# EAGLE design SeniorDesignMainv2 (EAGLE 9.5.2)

## Sheet 1 of 5: ESP32 Pinout and Power In ESP32 Device Pinout with connections to all other devices
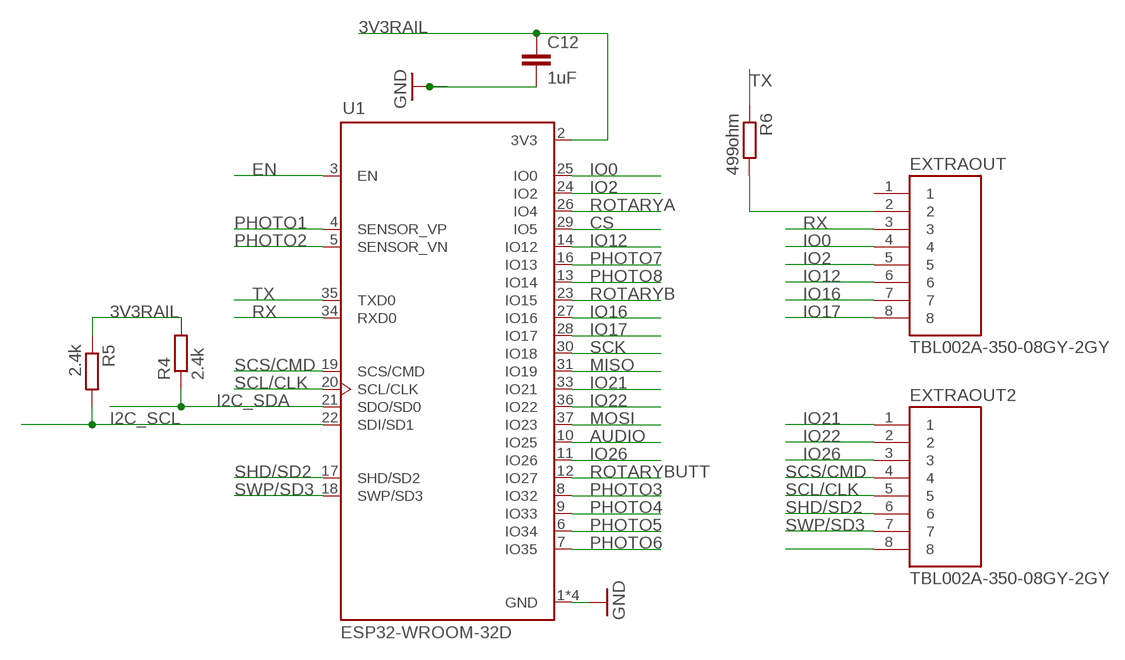
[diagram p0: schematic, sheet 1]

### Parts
C12  1uF  C-EUC1206  [C1206]
EXTRAOUT  TBL002A-350-08GY-2GY  [CUI_TBL002A-350-08GY-2GY]
EXTRAOUT2  TBL002A-350-08GY-2GY  [CUI_TBL002A-350-08GY-2GY]
R4  2.4k  R-EU_R1206  [R1206]
R5  2.4k  R-EU_R1206  [R1206]
R6  499ohm  R-EU_R1206  [R1206]
U1  ESP32-WROOM-32D  [MODULE_ESP32-WROOM-32D]

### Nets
3V3RAIL: C12.1 R4.2 R5.1 U1.2(3V3) ; also sheet 2,4,5
AUDIO: U1.10(IO25) ; also sheet 3
CS: U1.29(IO5) ; also sheet 5
EN: U1.3(EN)
GND: C12.2 U1.1(GND) U1.15(GND) U1.38(GND) U1.39(GND) ; also sheet 2,3,4,5
I2C_SCL: R5.2 U1.22(SDI/SD1) ; also sheet 5
I2C_SDA: R4.1 U1.21(SDO/SD0) ; also sheet 5
IO0: EXTRAOUT.4 U1.25(IO0)
IO2: EXTRAOUT.5 U1.24(IO2)
IO12: EXTRAOUT.6 U1.14(IO12)
IO16: EXTRAOUT.7 U1.27(IO16)
IO17: EXTRAOUT.8 U1.28(IO17)
IO21: EXTRAOUT2.1 U1.33(IO21)
IO22: EXTRAOUT2.2 U1.36(IO22)
IO26: EXTRAOUT2.3 U1.11(IO26)
MISO: U1.31(IO19) ; also sheet 5
MOSI: U1.37(IO23) ; also sheet 5
N$8: EXTRAOUT.2 R6.2
N$12: EXTRAOUT2.8
PHOTO1: U1.4(SENSOR_VP) ; also sheet 4
PHOTO2: U1.5(SENSOR_VN) ; also sheet 4
PHOTO3: U1.8(IO32) ; also sheet 4
PHOTO4: U1.9(IO33) ; also sheet 4
PHOTO5: U1.6(IO34) ; also sheet 4
PHOTO6: U1.7(IO35) ; also sheet 4
PHOTO7: U1.16(IO13) ; also sheet 4
PHOTO8: U1.13(IO14) ; also sheet 4
ROTARYA: U1.26(IO4) ; also sheet 5
ROTARYB: U1.23(IO15) ; also sheet 5
ROTARYBUTT: U1.12(IO27) ; also sheet 5
RX: EXTRAOUT.3 U1.34(RXD0)
SCK: U1.30(IO18) ; also sheet 5
SCL/CLK: EXTRAOUT2.5 U1.20(SCL/CLK)
SCS/CMD: EXTRAOUT2.4 U1.19(SCS/CMD)
SHD/SD2: EXTRAOUT2.6 U1.17(SHD/SD2)
SWP/SD3: EXTRAOUT2.7 U1.18(SWP/SD3)
TX: R6.1 U1.35(TXD0)
Unconnected: EXTRAOUT.1

## Sheet 2 of 5: Power/Voltage Regulators Basic/per data sheet setups for all the voltage regulators
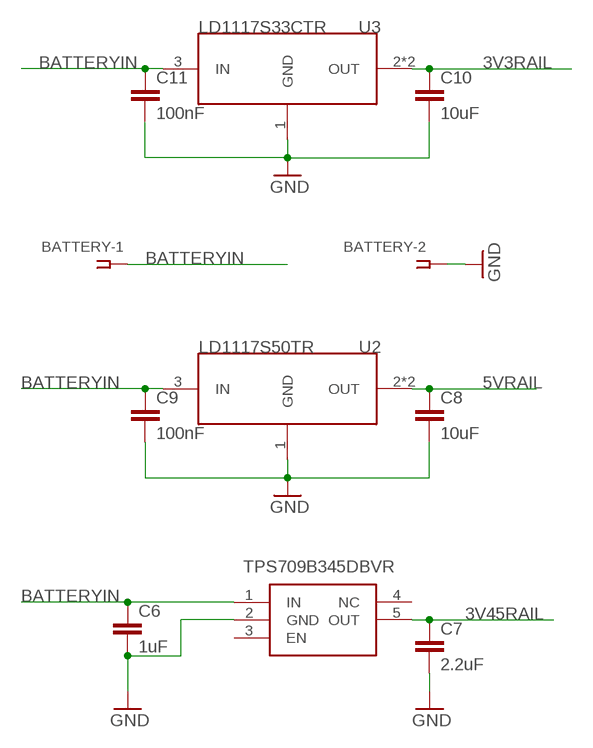
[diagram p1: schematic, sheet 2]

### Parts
BATTERY  SSW-101-02-G-D  [SSW-101-02-G-D]
C6  1uF  C-EUC1206  [C1206]
C7  2.2uF  C-EUC1206  [C1206]
C8  10uF  C-EUC1206  [C1206]
C9  100nF  C-EUC1206  [C1206]
C10  10uF  C-EUC1206  [C1206]
C11  100nF  C-EUC1206  [C1206]
IC1  TPS709B345DBVR  [SOT95P280X145-5N]
U2  LD1117S50TR  [SOT223]
U3  LD1117S33CTR  [SOT223]

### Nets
3V3RAIL: C10.1 U3.2(OUT) U3.4(OUT) ; also sheet 1,4,5
3V45RAIL: C7.1 IC1.5(OUT) ; also sheet 4
5VRAIL: C8.1 U2.2(OUT) U2.4(OUT) ; also sheet 3,5
BATTERYIN: BATTERY.1 C6.1 C9.1 C11.1 IC1.1(IN) U2.3(IN) U3.3(IN)
GND: BATTERY.2 C6.2 C7.2 C8.2 C9.2 C10.2 C11.2 IC1.2(GND) U2.1(GND) U3.1(GND) ; also sheet 1,3,4,5
Unconnected: IC1.3(EN) IC1.4(NC)

## Sheet 3 of 5: Audio Circuit LM 386 with Bass Boost Requires: 5 Capacitors, 3 Resistors, 4 Mount Holes
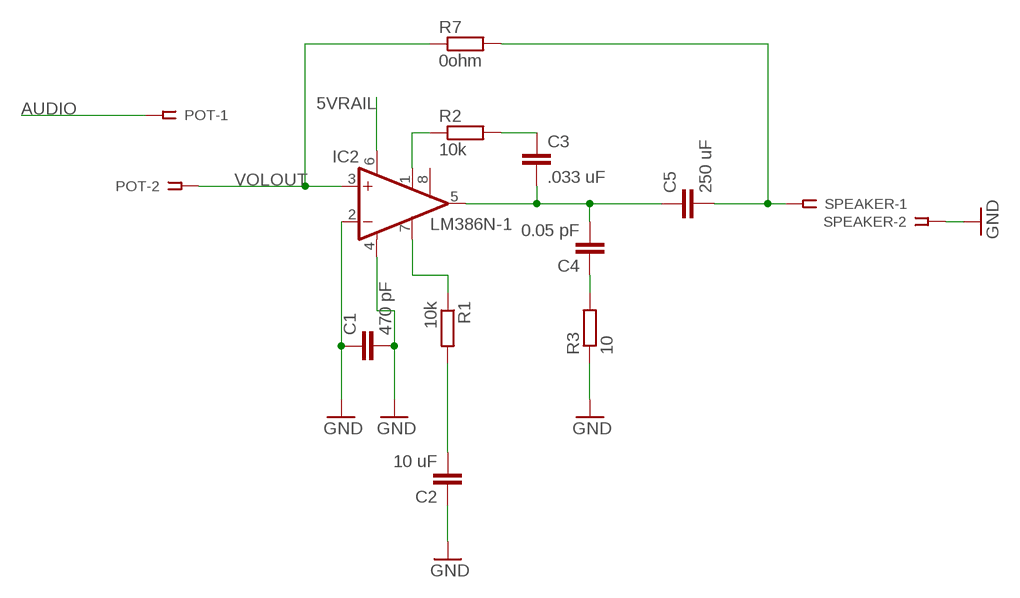
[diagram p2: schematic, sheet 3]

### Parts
C1  470 pF  C-EUC1206  [C1206]
C2  10 uF  C-EUC1206  [C1206]
C3  .033 uF  C-EUC1206  [C1206]
C4  0.05 pF  C-EUC1206  [C1206]
C5  250 uF  C-EUC1206  [C1206]
IC2  LM386N-1  [DIL08]
POT  SSW-101-02-G-D  [SSW-101-02-G-D]
R1  10k  R-EU_R1206  [R1206]
R2  10k  R-EU_R1206  [R1206]
R3  10  R-EU_R1206  [R1206]
R7  0ohm  R-EU_R1206  [R1206]
SPEAKER  SSW-101-02-G-D  [SSW-101-02-G-D]

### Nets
5VRAIL: IC2.6(VS) ; also sheet 2,5
AUDIO: POT.1 ; also sheet 1
GND: C1.1 C1.2 C2.1 IC2.2(-IN) IC2.4(GND) R3.1 SPEAKER.2 ; also sheet 1,2,4,5
N$1: IC2.7(BYPASS) R1.1
N$2: C2.2 R1.2
N$3: IC2.1(GAIN) R2.1
N$4: C3.2 C4.2 C5.1 IC2.5(OUT)
N$5: C3.1 R2.2
N$6: C4.1 R3.2
N$7: C5.2 R7.2 SPEAKER.1
VOLOUT: IC2.3(+IN) POT.2 R7.1
Unconnected: IC2.8(GAIN)

## Sheet 4 of 5: Laser Diodes and Photo Transistors Mapping from MCU to ports for the laser diodes. Mapping from MCU to ports for the phototransistors. WARNING: MCU LINES AND PORT HOLES ARE 1 INDEXED Extra Terminal for ground connections
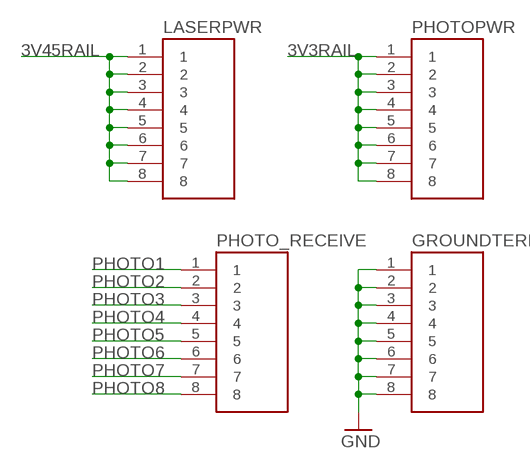
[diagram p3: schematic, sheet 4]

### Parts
GROUNDTERM  TBL002A-350-08GY-2GY  [CUI_TBL002A-350-08GY-2GY]
LASERPWR  TBL002A-350-08GY-2GY  [CUI_TBL002A-350-08GY-2GY]
PHOTO_RECEIVE  TBL002A-350-08GY-2GY  [CUI_TBL002A-350-08GY-2GY]
PHOTOPWR  TBL002A-350-08GY-2GY  [CUI_TBL002A-350-08GY-2GY]

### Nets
3V3RAIL: PHOTOPWR.1 PHOTOPWR.2 PHOTOPWR.3 PHOTOPWR.4 PHOTOPWR.5 PHOTOPWR.6 PHOTOPWR.7 PHOTOPWR.8 ; also sheet 1,2,5
3V45RAIL: LASERPWR.1 LASERPWR.2 LASERPWR.3 LASERPWR.4 LASERPWR.5 LASERPWR.6 LASERPWR.7 LASERPWR.8 ; also sheet 2
GND: GROUNDTERM.1 GROUNDTERM.2 GROUNDTERM.3 GROUNDTERM.4 GROUNDTERM.5 GROUNDTERM.6 GROUNDTERM.7 GROUNDTERM.8 ; also sheet 1,2,3,5
PHOTO1: PHOTO_RECEIVE.1 ; also sheet 1
PHOTO2: PHOTO_RECEIVE.2 ; also sheet 1
PHOTO3: PHOTO_RECEIVE.3 ; also sheet 1
PHOTO4: PHOTO_RECEIVE.4 ; also sheet 1
PHOTO5: PHOTO_RECEIVE.5 ; also sheet 1
PHOTO6: PHOTO_RECEIVE.6 ; also sheet 1
PHOTO7: PHOTO_RECEIVE.7 ; also sheet 1
PHOTO8: PHOTO_RECEIVE.8 ; also sheet 1

## Sheet 5 of 5: SPI to SD, I2C to LCD SD - Routing the MCU to communicate to the SD Card Reader via SPI potocol. The connection seen here is to a 7 pin header that will be on the board. This is the connection point for the breakout board and the MCU. LCD - 4 Pin Header. This could be to either a module for I2C or the chip if it's an issue to use the I2C module. 5 V are needed for the module and LCD. The 5 V Rail could be a direct connection from 5 V regulator or it could be from this pin.
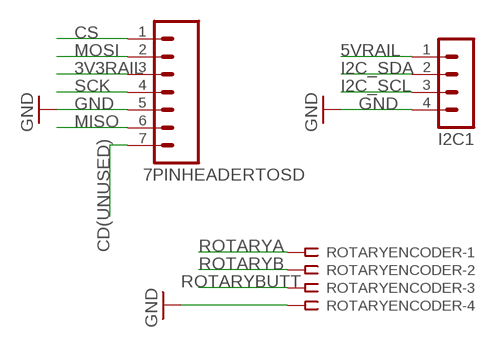
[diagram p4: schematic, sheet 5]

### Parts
7PINHEADERTOSD  M07  [07P]
I2C1  MA04-1  [MA04-1]
ROTARYENCODER  SSW-104-02-G-S  [SSW-104-02-G-S]

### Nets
3V3RAIL: 7PINHEADERTOSD.3 ; also sheet 1,2,4
5VRAIL: I2C1.1 ; also sheet 2,3
CD(UNUSED): 7PINHEADERTOSD.7
CS: 7PINHEADERTOSD.1 ; also sheet 1
GND: 7PINHEADERTOSD.5 I2C1.4 ROTARYENCODER.4 ; also sheet 1,2,3,4
I2C_SCL: I2C1.3 ; also sheet 1
I2C_SDA: I2C1.2 ; also sheet 1
MISO: 7PINHEADERTOSD.6 ; also sheet 1
MOSI: 7PINHEADERTOSD.2 ; also sheet 1
ROTARYA: ROTARYENCODER.1 ; also sheet 1
ROTARYB: ROTARYENCODER.2 ; also sheet 1
ROTARYBUTT: ROTARYENCODER.3 ; also sheet 1
SCK: 7PINHEADERTOSD.4 ; also sheet 1

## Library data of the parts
7PINHEADERTOSD = con-amp-quick:M07: AMP QUICK CONNECTOR; OC_FARNELL: unknown; OC_NEWARK: unknown
BATTERY POT SPEAKER = con-samtec:SSW-101-02-G: THROUGH-HOLE .025" SQ POST SOCKET; MF: Samtec Inc.; MPN: SSW-101-02-G-D; OC_FARNELL: unknown; OC_NEWARK: 82P1456
C1-C12 = rcl:C-EU: CAPACITOR, European symbol; SPICEPREFIX: C
EXTRAOUT EXTRAOUT2 GROUNDTERM LASERPWR PHOTO_RECEIVE PHOTOPWR = TBL002A-350-08GY-2GY:TBL002A-350-08GY-2GY; AVAILABILITY: Unavailable; CUI_PURCHASE_URL: https://www.cuidevices.com/product/interconnect/connectors/terminal-blocks/tbl002a-350-series?utm_source=snapeda.com&utm_medium=referral&utm_campaign=snapedaBOM; DESCRIPTION: 1~24 Poles, Screwless, 45°, 3.50 Pitch, 24~20 _AWG_, Terminal Block Connector; MF: CUI Devices; MP: TBL002A-350-08GY-2GY; PACKAGE: None; PRICE: None
I2C1 = con-lstb:MA04-1: PIN HEADER; OC_FARNELL: unknown; OC_NEWARK: unknown
IC1 = SamacSys_Parts:TPS709B345DBVR: LDO Voltage Regulators TPS709 DIE IN TLV704 PINOUT Source: Datasheet; DESCRIPTION: LDO Voltage Regulators TPS709 DIE IN TLV704 PINOUT; HEIGHT: 1.45mm; MANUFACTURER_NAME: Texas Instruments; MANUFACTURER_PART_NUMBER: TPS709B345DBVR
IC2 = linear:LM386?-*: Low Voltage Audio Power Amplifier Source: http://cache.national.com/ds/LM/LM386.pdf
R1-R7 = rcl:R-EU_: RESISTOR, European symbol; SPICEPREFIX: R
ROTARYENCODER = con-samtec:SSW-104-02-G-S: THROUGH-HOLE .025" SQ POST SOCKET Source: Samtec SSW.pdf; MF: Samtec Inc.; MPN: SSW-104-02-G-S; OC_FARNELL: unknown; OC_NEWARK: 11P9384
U1 = ESP32-WROOM-32D:ESP32-WROOM-32D: IC: SoC; GPIO, I2C, I2S, IR, SD, SDIO, SPI, UART; 2.7÷3.6VDC; 20dBm; AVAILABILITY: Unavailable; DESCRIPTION: Bluetooth, WiFi 802.11b/g/n, Bluetooth v4.2 + EDR, Class 1, 2 and 3 Transceiver Module 2.4GHz ~ 2.5GHz Integrated, Trace Surface Mount; MF: Espressif Systems; MP: ESP32-WROOM-32D; PACKAGE: Module Espressif Systems; PRICE: None
U2 = LD1117S50TR:LD1117S50TR: http://octopart.com/ld1117s50tr-stmicroelectronics-529395; AVAILABILITY: Unavailable; DESCRIPTION: Linear Voltage Regulator IC 1 Output 800mA SOT-223; MF: STMicroelectronics; MP: LD1117S50TR; PACKAGE: SOT-223 STMicroelectronics; PRICE: None
U3 = LD1117S33CTR:LD1117S33CTR: http://octopart.com/ld1117s33tr-stmicroelectronics-526708; AVAILABILITY: Unavailable; DESCRIPTION: Linear Voltage Regulator IC 1 Output 800mA SOT-223; MF: STMicroelectronics; MP: LD1117S33CTR; PACKAGE: SOT-223 STMicroelectronics; PRICE: None

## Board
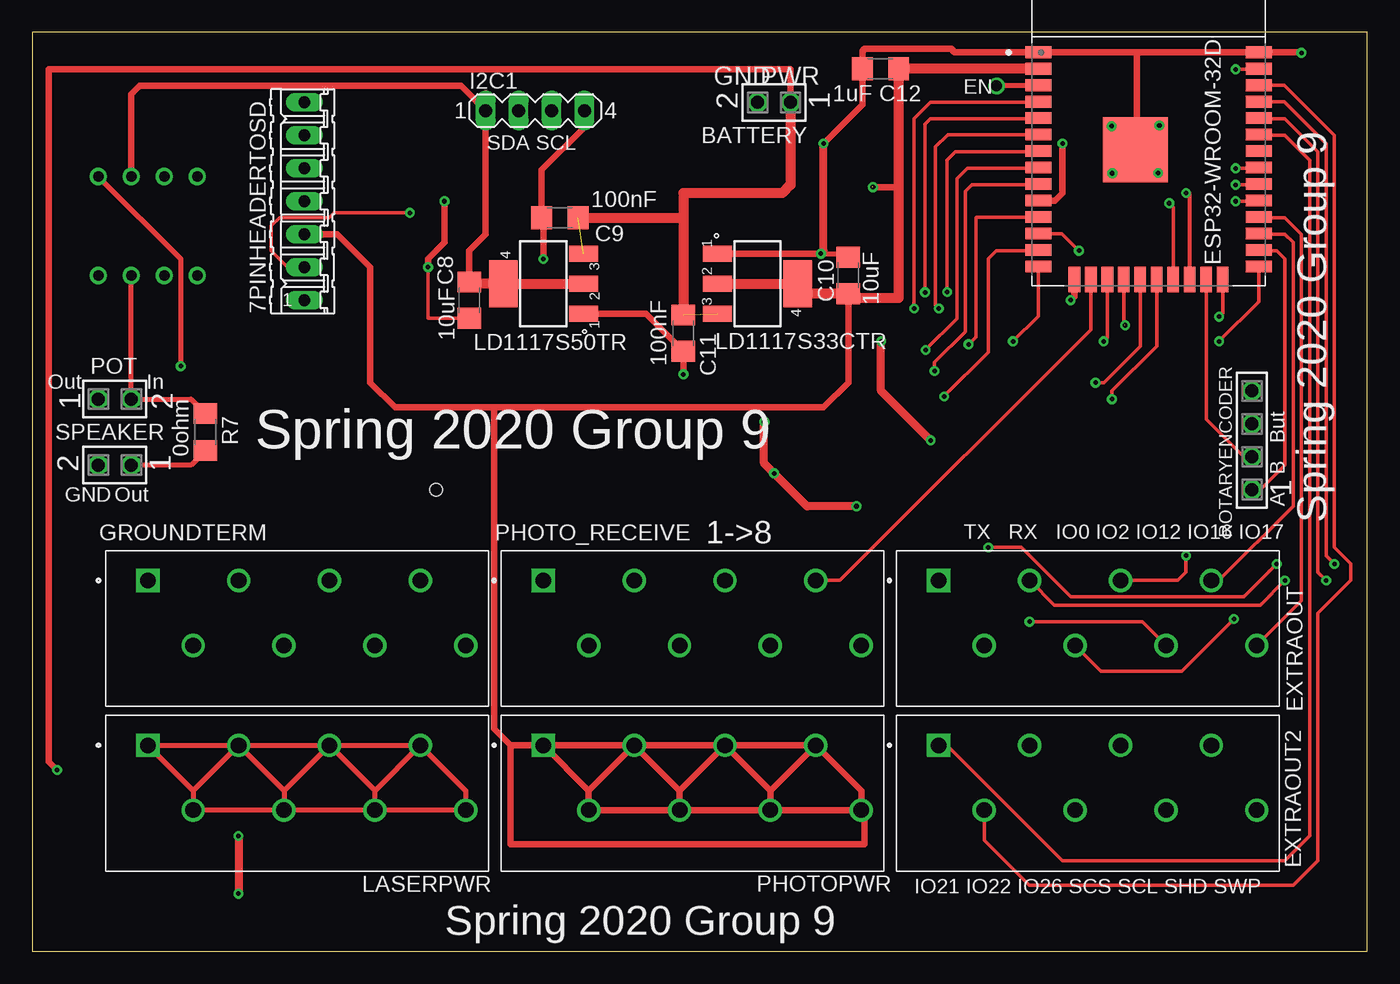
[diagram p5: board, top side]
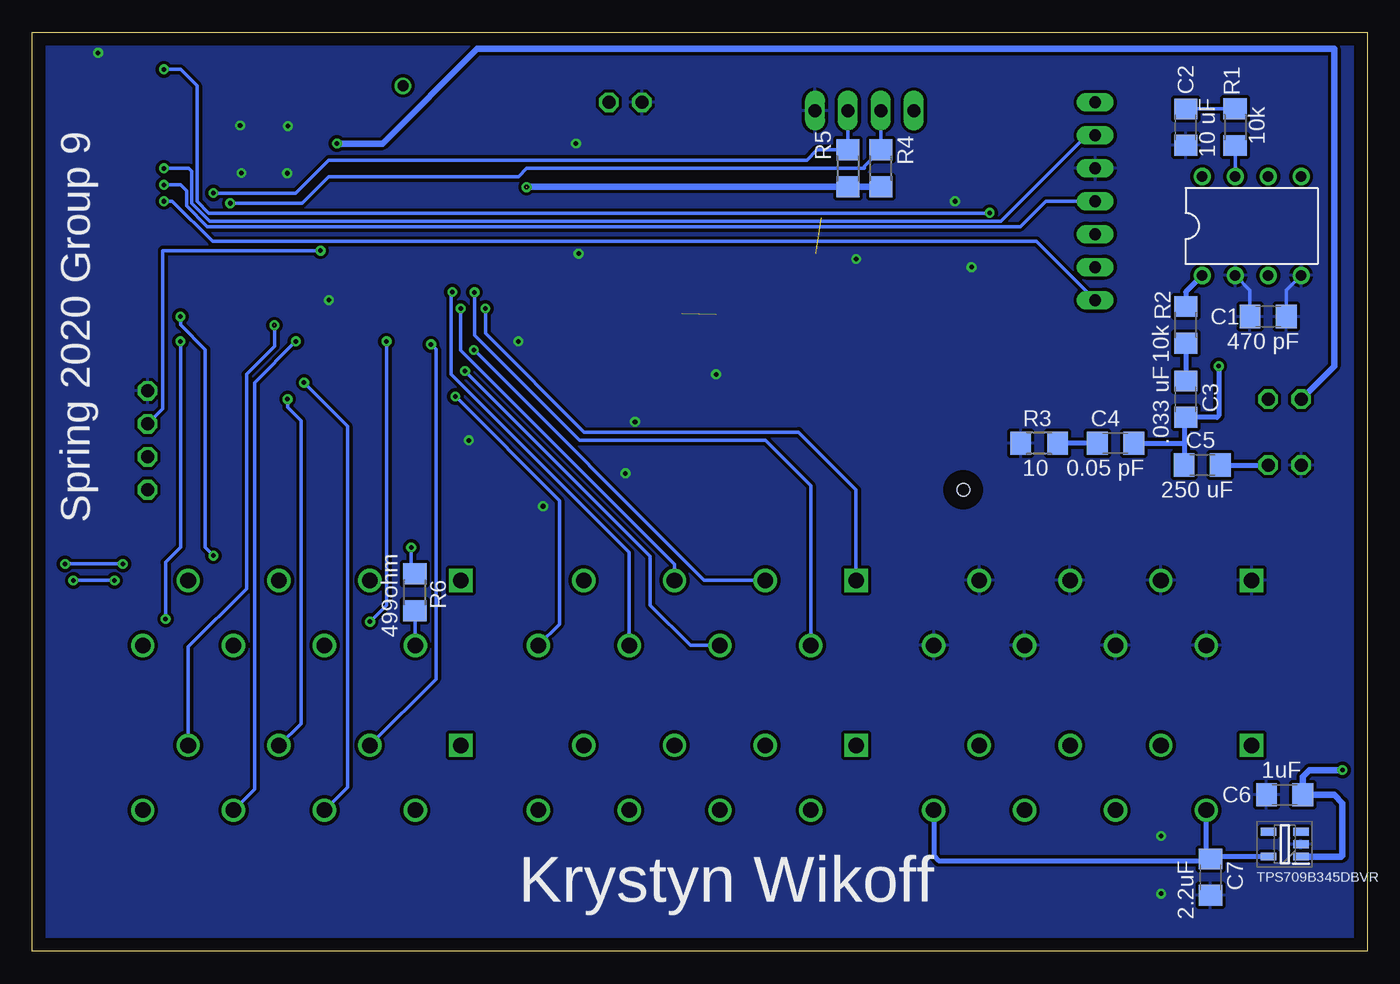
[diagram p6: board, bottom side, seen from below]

Size 102.85 x 70.79 mm. Coordinates in mm from the lower left corner, seen from the top.
Outline: 0,0 102.85,0 102.85,70.79 0,70.79 0,0
Copper layers (1*16): Top 0.035mm / dielectric 1.5mm / Bottom 0.035mm
Design rules "default": minimum track width 6mil, minimum drill 0.35mm, track to track 6mil, track to pad 6mil, pad to pad 6mil, via to via 6mil, smd to smd 6mil, copper to edge 40mil, drill to drill 6mil, minimum pad ring 10mil, minimum via ring 8mil, stop-mask expansion 4mil, vias tented up to drill 0mil, thermal gap 10mil
Holes 1 mm at 31.11,35.56

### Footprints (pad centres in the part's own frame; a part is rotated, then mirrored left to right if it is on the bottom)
07P = drill 0.914 long: 1 -7.62,0; 2 -5.08,0; 3 -2.54,0; 4 0,0; 5 2.54,0; 6 5.08,0; 7 7.62,0
SSW-101-02-G-D = drill 1 pad 1.5 octagon: 1 0,-1.27; 2 0,1.27
C1206 = smd 1.6 x 1.8: 1 -1.4,0; 2 1.4,0
CUI_TBL002A-350-08GY-2GY = drill 1.2 square: 1 0,0 | drill 1.2: 2 3.5,-5; 3 7,0; 4 10.5,-5; 5 14,0; 6 17.5,-5; 7 21,0; 8 24.5,-5
MA04-1 = drill 1.016 long: 1 -3.81,0; 2 -1.27,0; 3 1.27,0; 4 3.81,0
SOT95P280X145-5N = smd 1.2 x 0.6: 1 -1.25,0.95; 2 -1.25,0; 3 -1.25,-0.95; 4 1.25,-0.95; 5 1.25,0.95
DIL08 = drill 0.813 pad 1.27: 1 -3.81,-3.81; 2 -1.27,-3.81; 3 1.27,-3.81; 4 3.81,-3.81; 5 3.81,3.81; 6 1.27,3.81; 7 -1.27,3.81; 8 -3.81,3.81
R1206 = smd 1.6 x 1.803: 1 -1.422,0; 2 1.422,0
SSW-104-02-G-S = drill 1 pad 1.5 octagon: 1 -3.81,0; 2 -1.27,0; 3 1.27,0; 4 3.81,0
MODULE_ESP32-WROOM-32D = smd 2 x 0.9: 1 -8.5,5.26; 2 -8.5,3.99; 3 -8.5,2.72; 4 -8.5,1.45; 5 -8.5,0.18; 6 -8.5,-1.09; 7 -8.5,-2.36; 8 -8.5,-3.63; 9 -8.5,-4.9; 10 -8.5,-6.17; 11 -8.5,-7.44; 12 -8.5,-8.71; 13 -8.5,-9.98; 14 -8.5,-11.25; 25 8.5,-11.25; 26 8.5,-9.98; 27 8.5,-8.71; 28 8.5,-7.44; 29 8.5,-6.17; 30 8.5,-4.9; 31 8.5,-3.63; 32 8.5,-2.36; 33 8.5,-1.09; 34 8.5,0.18; 35 8.5,1.45; 36 8.5,2.72; 37 8.5,3.99; 38 8.5,5.26 | smd 0.9 x 2: 15 -5.715,-12.25; 16 -4.445,-12.25; 17 -3.175,-12.25; 18 -1.905,-12.25; 19 -0.635,-12.25; 20 0.635,-12.25; 21 1.905,-12.25; 22 3.175,-12.25; 23 4.445,-12.25; 24 5.715,-12.25 | smd 5 x 5: 39 -1,-2.24
SOT223 = smd 2.235 x 1.219: 1 -3.099,2.311; 2 -3.099,0; 3 -3.099,-2.311 | smd 2.2 x 3.6: 4 3.099,0

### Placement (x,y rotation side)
7PINHEADERTOSD  20.95,57.78 90 top
BATTERY  57.15,65.41 90 top
C1  7.62,48.9 0 bottom
C2  13.97,63.5 90 bottom
C3  13.97,42.55 270 bottom
C4  19.38,39.14 0 bottom
C5  12.7,37.47 0 bottom
C6  6.35,12.06 180 bottom
C7  12.06,5.71 270 bottom
C8  33.66,50.16 270 top
C9  40.64,56.52 180 top
C10  62.87,52.07 90 top
C11  50.16,47.62 270 top
C12  65.35,68 180 top
EXTRAOUT  69.85,28.57 0 top
EXTRAOUT2  69.85,15.88 0 top
GROUNDTERM  8.89,28.57 0 top
I2C1  38.73,64.77 0 top
IC1  6.35,8.26 180 bottom
IC2  8.89,55.88 0 bottom
LASERPWR  8.89,15.88 0 top
PHOTO_RECEIVE  39.37,28.57 0 top
PHOTOPWR  39.37,15.88 0 top
POT  6.35,42.55 270 top
R1  10.16,63.5 90 bottom
R2  13.97,48.26 270 bottom
R3  25.27,39.14 0 bottom
R4  37.47,60.33 270 bottom
R5  40.01,60.33 90 bottom
R6  73.38,27.66 270 bottom
R7  13.34,40.01 270 top
ROTARYENCODER  93.98,39.37 90 top
SPEAKER  6.35,37.47 90 top
U1  86,64.01 0 top
U2  39.37,51.44 180 top
U3  55.88,51.44 0 top

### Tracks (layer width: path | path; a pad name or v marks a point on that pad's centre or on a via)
3V3RAIL  (via drill 0.35)  (1 unrouted)
  Top 0.508: C10.1 62.87,43.81 60.96,41.91 35.56,41.91 | 35.56,41.91 35.56,17.14 36.83,15.88 | 36.83,15.88 PHOTOPWR.1 | PHOTOPWR.1 PHOTOPWR.3 | PHOTOPWR.3 PHOTOPWR.5 | PHOTOPWR.5 PHOTOPWR.7 | PHOTOPWR.1 42.87,12.38 | 42.87,12.38 PHOTOPWR.2 PHOTOPWR.4 | 42.87,12.38 PHOTOPWR.3 | PHOTOPWR.3 49.87,12.38 | PHOTOPWR.4 49.87,12.38 | 49.87,12.38 PHOTOPWR.5 | PHOTOPWR.7 56.87,12.38 | PHOTOPWR.5 56.87,12.38 | 56.87,12.38 PHOTOPWR.6 | PHOTOPWR.7 63.87,12.38 PHOTOPWR.8 | PHOTOPWR.8 PHOTOPWR.6 | PHOTOPWR.6 PHOTOPWR.4 | 36.83,15.88 36.83,8.26 64.14,8.26 64.14,10.61 PHOTOPWR.8 | 35.56,41.91 27.94,41.91 26.04,43.81 26.04,52.7 23.5,55.24 7PINHEADERTOSD.3 | 66.63,58.29 66.75,58.42 | v64.77,58.88 66.7,58.88 66.75,58.83
  Top 0.762: U3.2 U3.4 58.98,50.88 59.19,50.67 C10.1 63.21,50.33 66.75,50.33 66.75,58.42 66.75,58.83 C12.1 U1.2
  Bottom 0.508: R4.2 R5.1 64.74,58.9 64.75,58.9
3V45RAIL
  Top 0.381: LASERPWR.3 LASERPWR.1 12.39,12.38 | LASERPWR.3 LASERPWR.5 | LASERPWR.5 LASERPWR.7 | LASERPWR.7 33.39,12.38 LASERPWR.8 LASERPWR.6 | LASERPWR.6 LASERPWR.4 | LASERPWR.4 LASERPWR.2 12.39,12.38 | LASERPWR.3 12.39,12.38 | LASERPWR.3 19.39,12.38 | LASERPWR.5 19.39,12.38 | 19.39,12.38 LASERPWR.4 | LASERPWR.5 26.39,12.38 | LASERPWR.6 26.39,12.38 | 26.39,12.38 LASERPWR.7
  Bottom 0.381: IC1.5 11.88,7.3 C7.1 | C7.1 12.39,7.44 LASERPWR.2 | LASERPWR.8 33.39,7.36 33.02,6.99 12.2,6.99 C7.1
5VRAIL
  Top 0.508: C8.1 33.66,53.98 34.92,55.24 I2C1.1 33.02,66.67 8.26,66.67 7.62,66.04 IC2.6
  Top 0.635: I2C1.1 34.92,66.04
  Top 0.762: U2.2 U2.4 33.78,51.44 C8.1
AUDIO  (via drill 0.35)
  Top 0.508: 77.45,57.78 U1.10 78.79,57.84 79.38,58.42 v79.38,62.23
  Bottom 0.508: POT.1 2.54,45.09 2.54,69.52 68.58,69.52 75.87,62.23 v79.38,62.23
BATTERYIN  (via drill 0.35)  (2 unrouted)
  Top 0.508: BATTERY.1 58.42,67.94 1.27,67.94 1.27,14.61 v1.91,13.97
  Top 0.762: BATTERY.1 58.42,59.05 57.78,58.42 50.16,58.42 50.16,56.52 | 50.16,56.52 C11.1 | C9.1 50.16,56.52
  Bottom 0.508: 4.45,12.06 C6.1 | IC1.1 5.08,7.29 1.98,7.29 1.91,7.37 1.91,11.43 2.54,12.06 C6.1 | v1.91,13.97 4.45,13.97 4.95,13.46 C6.1
CS  (via drill 0.35)
  Top 0.254: U1.29 94.45,57.78 v92.71,57.78
  Bottom 0.254: v92.71,57.78 92.08,57.78 88.98,54.69 25.48,54.69 7PINHEADERTOSD.1
EN  (via drill 0.85)
  Top 0.381: U1.3 77.45,66.67 v74.3,66.67
GND  (via drill 0.35)
  Top 0.254: v30.48,52.7 30.48,48.77 C8.2
  Top 0.381: C10.2 62.59,53.75 v60.76,53.75 60.96,53.95
  Top 0.508: 85.04,69.27 U1.1 71.07,69.27 70.81,69.52 64.14,69.52 63.95,69.34 C12.2 63.95,65.22 v60.96,62.23 | 85.04,69.27 85.09,69.22 85.09,61.85 U1.39 | 85.04,69.27 U1.38 97.74,69.27 v97.79,69.22 | v30.48,52.7 30.48,53.34 31.75,54.61 v31.75,57.78 | v39.37,53.34 39.37,56.38 C9.2 39.24,60.2 42.55,63.5 I2C1.4 | v50.16,44.45 C11.2 47.27,49.12 U2.1 | U3.1 v60.76,53.75 | U1.15 80.29,50.44 v80.01,50.16
  Top 0.635: 60.96,53.95 v60.96,62.23 | v69.22,39.37 65.41,43.18 v65.41,46.99 | v63.5,34.29 59.69,34.29 v57.15,36.83 56.39,37.59 56.39,40.82 | v15.88,8.89 v15.88,4.45
  Bottom 0.254: IC2.4 6.22,50.93 C1.2 | C1.1 9.02,50.93 IC2.2
  other vias: 83.16,63.58 83.21,59.94 86.84,63.63 86.74,59.97 56.41,40.79
  pour Bottom (isolate 0.254): 0,70.48 69.22,70.48 69.85,69.85 102.87,69.85 102.87,0 0,0
I2C_SCL  (via drill 0.35)
  Top 0.305: U1.22 89.18,58.42 v88.9,58.42
  Bottom 0.254: I2C1.3 R5.2 42.39,61.75 43.18,60.96 80.01,60.96 82.55,58.42 v88.9,58.42
I2C_SDA  (via drill 0.35)
  Top 0.254: v87.61,57.63 87.91,57.33 U1.21
  Bottom 0.254: I2C1.2 R4.1 38.73,60.48 38.73,60.33 64.77,60.33 65.41,59.69 80.01,59.69 82.07,57.63 v87.61,57.63
IO0  (via drill 0.35)
  Top 0.254: U1.25 94.5,50.05 v91.44,46.99 | v92.58,25.6 88.57,21.59 82.33,21.59 EXTRAOUT.4
  Bottom 0.254: v91.44,46.99 91.44,31.11 92.58,29.97 v92.58,25.6
IO2  (via drill 0.35)
  Top 0.254: U1.24 91.72,49.17 v91.44,48.9 | v88.9,30.48 88.9,29.21 88.27,28.57 EXTRAOUT.5
  Bottom 0.254: v91.44,48.9 91.44,48.26 89.53,46.35 89.53,31.11 v88.9,30.48
IO12  (via drill 0.35)
  Top 0.254: U1.14 77.5,48.93 v75.56,46.99 | EXTRAOUT.6 85.53,25.4 v76.83,25.4
  Bottom 0.254: v75.56,46.99 75.56,26.67 v76.83,25.4
IO16
  Top 0.254: U1.27 94.56,55.24 96.52,55.24 97.16,54.61 97.16,34.29 91.44,28.57 EXTRAOUT.7
IO17
  Top 0.254: U1.28 94.56,56.52 96.52,56.52 97.79,55.24 97.79,27.02 EXTRAOUT.8
IO21
  Top 0.254: U1.33 94.56,62.87 96.52,62.87 98.42,60.96 98.42,8.89 96.52,6.99 79.38,6.99 70.48,15.88 EXTRAOUT2.1
IO22
  Top 0.254: U1.36 96.47,66.73 100.33,62.87 100.33,31.11 101.6,29.84 101.6,28.57 99.06,26.04 99.06,6.99 97.16,5.08 76.83,5.08 73.35,8.56 EXTRAOUT2.2
IO26  (via drill 0.35)
  Top 0.254: U1.11 72.75,56.57 72.69,56.52 72.69,47.32 v72.14,46.76
  Bottom 0.254: EXTRAOUT2.3 71.75,20.97 71.75,46.38 v72.14,46.76
MISO  (via drill 0.35)
  Top 0.254: U1.31 94.45,60.33 v92.71,60.33
  Bottom 0.254: v92.71,60.33 90.81,60.33 90.58,60.1 90.58,57.62 89.2,56.24 28.22,56.24 21.59,62.87 7PINHEADERTOSD.6
MOSI  (via drill 0.35)
  Top 0.254: U1.37 94.45,67.94 v92.71,67.94 | v29.08,56.9 23.24,56.9 22.86,56.52 19.05,56.52 18.41,55.88 18.41,53.98 19.68,52.7 7PINHEADERTOSD.2
  Bottom 0.254: v92.71,67.94 91.44,67.94 90.17,66.67 90.17,57.78 89.26,56.87 29.11,56.87 v29.08,56.9
N$1
  Bottom 0.254: IC2.7 R1.1
N$2
  Bottom 0.254: R1.2 13.95,64.92 C2.2
N$3
  Bottom 0.381: IC2.1 13.97,50.8 R2.1
N$4  (via drill 0.35)
  Top 0.381: IC2.5 11.43,53.34 v11.43,45.09
  Bottom 0.381: 14.1,39.19 14.1,41.02 C3.2 11.56,41.15 11.43,41.27 v11.43,45.09 | 14.1,39.19 C5.1 | C4.2 14.15,39.14 14.1,39.19
N$5
  Bottom 0.381: R2.2 C3.1
N$6
  Bottom 0.381: C4.1 R3.2
N$7
  Top 0.381: R7.2 12.22,37.47 SPEAKER.1
  Bottom 0.381: C5.2 SPEAKER.1
N$8
  Bottom 0.254: R6.2 73.35,26.21 EXTRAOUT.2
PHOTO1  (via drill 0.35)
  Top 0.254: U1.4 77.45,65.41 69.22,65.41 67.94,64.14 v67.94,49.53
  Bottom 0.254: v67.94,49.53 67.94,47.62 60.33,40.01 43.81,40.01 39.37,35.56 PHOTO_RECEIVE.1
PHOTO2  (via drill 0.35)
  Top 0.254: U1.5 77.45,64.14 69.22,64.14 68.78,63.7 v68.78,50.77
  Bottom 0.254: v68.78,50.77 68.78,47.45 60.71,39.37 46.35,39.37 42.87,35.88 PHOTO_RECEIVE.2
PHOTO3  (via drill 0.35)
  Top 0.254: U1.8 77.45,60.33 72.06,60.33 71.25,59.51 71.25,48.74 v68.83,46.33
  Bottom 0.254: v68.83,46.33 51.08,28.57 PHOTO_RECEIVE.3
PHOTO4  (via drill 0.35)
  Top 0.254: U1.9 77.45,59.05 72.39,59.05 71.88,58.55 71.88,47.75 69.52,45.39 v69.52,44.7
  Bottom 0.254: v69.52,44.7 55.24,30.43 55.24,26.67 52.15,23.57 PHOTO_RECEIVE.4
PHOTO5  (via drill 0.35)
  Top 0.254: U1.6 70.54,62.92 69.6,61.98 69.6,49.78 v69.85,49.53
  Bottom 0.254: v69.85,49.53 69.85,46.3 53.37,29.82 PHOTO_RECEIVE.5
  other vias: 53.37,28.57
PHOTO6  (via drill 0.35)
  Top 0.254: U1.7 77.45,61.59 71.12,61.59 70.48,60.96 v70.48,50.8
  Bottom 0.254: v70.48,50.8 70.59,50.7 70.59,44.45 56.87,30.73 PHOTO_RECEIVE.6
PHOTO7
  Top 0.254: U1.16 81.56,47.9 62.23,28.57 PHOTO_RECEIVE.7
PHOTO8  (via drill 0.35)
  Top 0.254: U1.13 77.45,53.98 74.3,53.98 73.66,53.34 73.66,46.15 v70.26,42.75
  Bottom 0.254: v70.26,42.75 62.23,34.72 62.23,25.21 PHOTO_RECEIVE.8
ROTARYA
  Top 0.254: U1.26 94.56,53.98 95.89,53.98 96.52,53.34 96.52,37.47 94.61,35.56 ROTARYENCODER.1
ROTARYB
  Top 0.254: U1.23 90.45,41 93.34,38.1 ROTARYENCODER.2
ROTARYBUTT  (via drill 0.35)
  Top 0.254: U1.12 79.32,55.3 v80.64,53.98
  Bottom 0.254: v80.64,53.98 92.81,53.98 92.81,41.81 ROTARYENCODER.3
RX  (via drill 0.35)
  Top 0.254: U1.34 94.56,64.14 96.52,64.14 99.06,61.59 99.06,29.21 v99.69,28.57 | v96.52,28.57 94.61,26.67 78.75,26.67 EXTRAOUT.3
  Bottom 0.254: v99.69,28.57 v96.52,28.57
SCK  (via drill 0.35)
  Top 0.254: U1.30 94.45,59.05 v92.71,59.05
  Bottom 0.254: v92.71,59.05 91.44,59.05 90.98,58.6 90.98,57.45 89.37,55.83 26.72,55.83 24.77,57.78 7PINHEADERTOSD.4
SCL/CLK  (via drill 0.35)
  Top 0.254: U1.20 86.64,46.63 83.19,43.18 v83.19,42.55
  Bottom 0.254: v83.19,42.55 83.19,41.91 82.14,40.87 82.14,17.55 83.82,15.88 EXTRAOUT2.5
SCS/CMD  (via drill 0.35)
  Top 0.254: U1.19 85.37,46.63 82.55,43.81 v81.92,43.81
  Bottom 0.254: v81.92,43.81 78.57,40.47 78.57,12.65 EXTRAOUT2.4
SHD/SD2  (via drill 0.35)
  Top 0.254: U1.17 82.83,47.27 v82.55,46.99
  Bottom 0.254: v82.55,46.99 85.72,43.81 85.72,12.5 EXTRAOUT2.6
SWP/SD3  (via drill 0.35)  (1 unrouted)
  Top 0.254: U1.18 84.1,48.36 84.2,48.26
  Bottom 0.254: v84.2,48.23 84.2,46.61 86.36,44.45 86.36,27.94 90.85,23.45 EXTRAOUT2.7
TX  (via drill 0.35)
  Top 0.254: U1.35 96.47,65.46 99.69,62.23 99.69,30.48 v100.33,29.84 | v95.89,29.84 93.34,27.3 80.01,27.3 76.2,31.11 v73.66,31.11
  Bottom 0.254: v100.33,29.84 v95.89,29.84 | v73.66,31.11 73.66,29.36 R6.1
VOLOUT
  Top 0.381: IC2.3 POT.2 12.22,42.55 R7.1

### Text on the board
tNames: GND | PWR | EN | SDA SCL | Out | In | Spring 2020 Group 9 | GND | Out | A B But | Spring 2020 Group 9 | TX RX IO0 IO2 IO12 IO16 IO17 | 1->8 | IO21 IO22 IO26 SCS SCL SHD SWP | Spring 2020 Group 9
bNames: Spring 2020 Group 9 | Krystyn Wikoff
